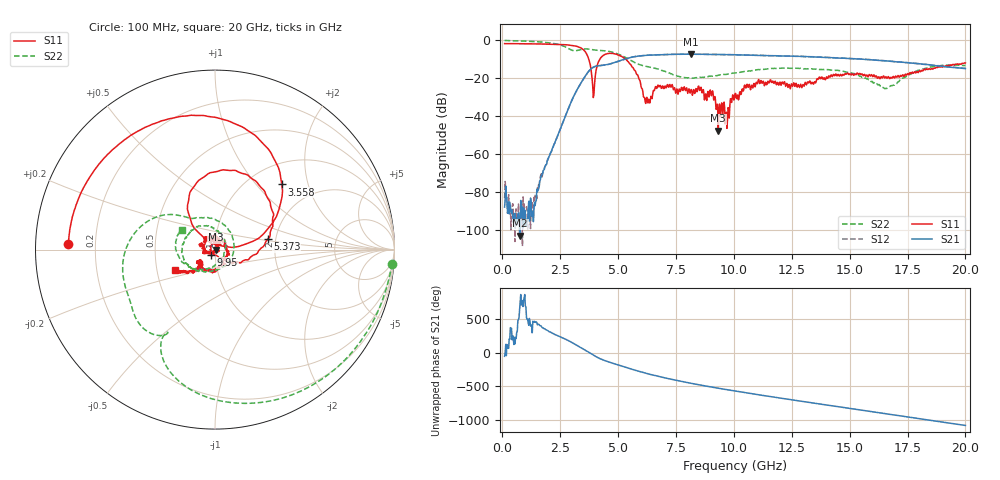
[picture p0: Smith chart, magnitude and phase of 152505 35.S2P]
!  2-Port S-parameters saved by WinCal
! VAR MeasName=S-Parameters (CALIBRATED_DATA) read from VNA (N5230C)
! VAR MeasDate=4/10/2015 9:31:58 AM
! VAR NAME=152505 35
! VAR FILENAME=152505 35.S2P
! VAR DATE=4/10/2015 9:31:58 AM
! VAR PHYS_PORTS=1,2
# Hz S DB R 50
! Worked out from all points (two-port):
!   801 points, 100 MHz to 20 GHz, reference 50 ohm
!   highest |S21| = -7.30 dB at 8.159 GHz (marker M1); lowest = -102.9 dB at 771.6 MHz (marker M2)
!   |S21| within 3 dB of the highest: 5.192 GHz to 15.94 GHz (10.75 GHz wide, 102 % of centre); 15.96237 GHz to 15.9734 GHz (11.03 MHz wide, 0.0691 % of centre)
!   lowest |S11| = -47.6 dB at 9.329 GHz (marker M3), VSWR 1.01, Z = 50.4 + j0.00173 ohm
!   |S11| at or under -10 dB: 3.735 GHz to 4.21 GHz (475.1 MHz wide, 12 % of centre); 5.328 GHz to end of sweep
!   |S22| runs from -25.5 to -0.1 dB; largest |S21 - S12| = 0.0052
!   S11 on the Smith chart (normalised r, x): 100 MHz: 0.10, +0.02; 3.558 GHz: 1.39, +1.38; 5.373 GHz: 1.81, +0.23; 9.95 GHz: 0.96, -0.06; 20 GHz: 0.62, -0.15
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1e8  -1.75 177.6  -87.83 -54.1  -83.08 -44.8  -0.09 -4.5
7.71625e8  -1.81 161.6  -102.92 37.8  -97.85 56.5  -0.35 -31.3
1.493e9  -1.91 143.5  -78.48 89.0  -83.28 105.9  -0.74 -60.8
2.5875e9  -2.25 109.0  -44.18 -136.3  -44.27 -137.0  -2.78 -110.1
3.43325e9  -4.31 57.9  -21.75 68.5  -21.76 68.9  -4.78 -124.3
3.557625e9  -5.69 44.3  -19.31 44.3  -19.32 44.5  -4.56 -129.6
3.93075e9  -30.14 52.1  -14.18 -35.8  -14.18 -35.6  -5.03 -146.3
4.3785e9  -7.88 100.5  -13.08 -111.5  -13.12 -111.7  -5.49 -164.2
5.3735e9  -10.50 11.2  -9.60 137.6  -9.57 137.6  -9.42 145.0
6.194375e9  -33.24 -133.6  -7.92 54.3  -7.91 54.1  -13.64 122.4
6.741625e9  -23.70 116.0  -7.62 7.3  -7.62 7.0  -15.18 95.1
8.1595e9  -25.89 92.3  -7.30 -95.9  -7.31 -95.9  -19.91 -31.0
9.00525e9  -27.37 61.1  -7.45 -149.8  -7.43 -149.6  -18.86 -86.7
9.328625e9  -47.58 0.2  -7.46 -169.0  -7.50 -169.2  -18.38 -96.3
9.726625e9  -41.66 -138.1  -7.57 167.8  -7.55 167.8  -17.81 -109.7
9.9505e9  -28.77 -125.4  -7.59 154.9  -7.60 154.8  -17.31 -114.5
1.005e10  -28.15 -132.4  -7.61 149.2  -7.64 149.1  -17.20 -117.4
1.146788e10  -21.56 131.7  -8.08 72.3  -8.03 72.4  -15.00 -153.7
1.338325e10  -22.11 -30.1  -8.72 -26.7  -8.67 -26.5  -15.08 158.5
1.477625e10  -18.11 -117.9  -9.46 -97.5  -9.43 -97.8  -16.43 118.7
1.669162e10  -19.40 -134.2  -10.95 164.9  -10.95 164.2  -24.45 -34.8
2e10  -11.95 -153.0  -14.90 -3.0  -14.86 -2.9  -13.35 149.3
